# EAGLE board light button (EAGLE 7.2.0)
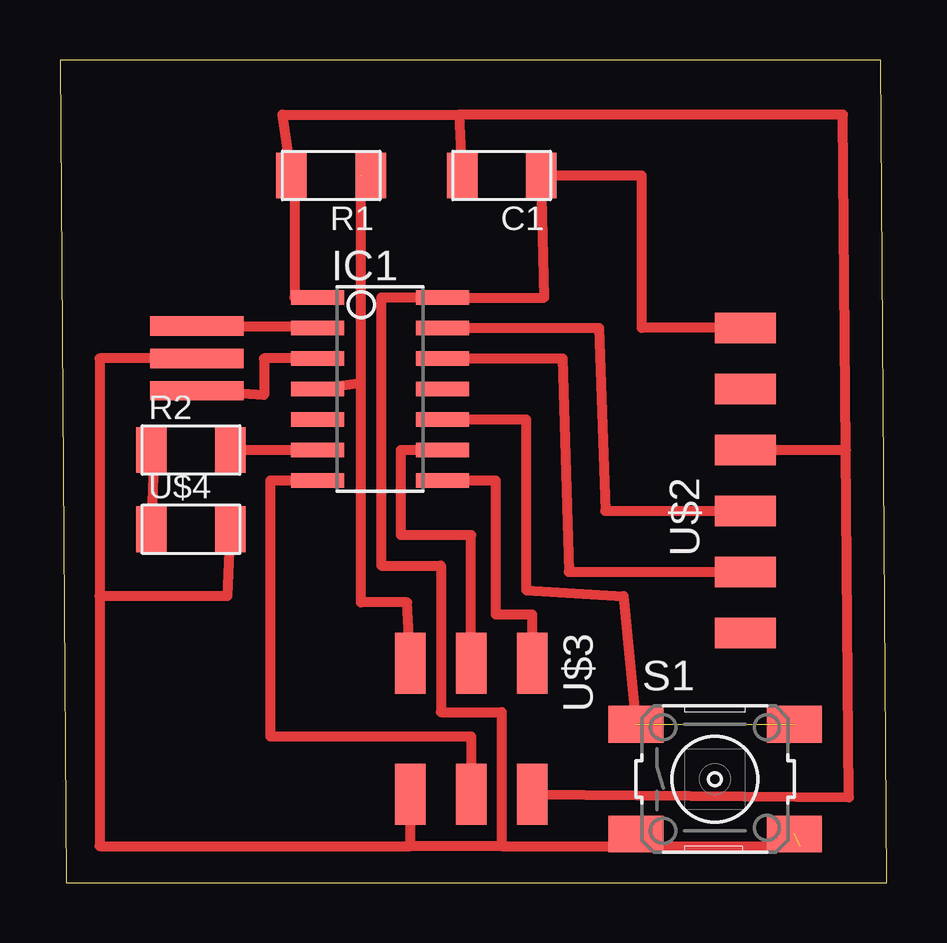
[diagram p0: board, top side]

Size 34.47 x 34.28 mm. Coordinates in mm from the lower left corner, seen from the top.
Outline: 0.25,0 34.47,0 34.21,34.28 0,34.28 0.25,0
Copper layers (1*16): Top 0.035mm / dielectric 1.5mm / Bottom 0.035mm
Design rules "default *": minimum track width 10mil, minimum drill 24mil, track to track 0.41mm, track to pad 0.41mm, pad to pad 0.41mm, via to via 0.41mm, smd to smd 8mil, copper to edge 40mil, drill to drill 8mil, minimum pad ring 10mil, minimum via ring 8mil, stop-mask expansion 4mil, vias tented up to drill 0mil, thermal gap 10mil

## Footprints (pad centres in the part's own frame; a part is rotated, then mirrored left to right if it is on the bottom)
C1206FAB = smd 1.27 x 1.905: 1 -1.651,0; 2 1.651,0
SOIC14 = smd 0.61 x 2.21: 1 -3.81,-2.603; 2 -2.54,-2.603; 3 -1.27,-2.603; 4 0,-2.603; 5 1.27,-2.603; 6 2.54,-2.603; 7 3.81,-2.603; 8 3.81,2.603; 9 2.54,2.603; 10 1.27,2.603; 11 0,2.603; 12 -1.27,2.603; 13 -2.54,2.603; 14 -3.81,2.603
R1206FAB = smd 1.27 x 1.905: 1 -1.651,0; 2 1.651,0
6MM_SWITCH = smd 2.286 x 1.524: 1 -3.302,2.286; 2 3.302,2.286; 3 -3.302,-2.286; 4 3.302,-2.286
EFOBM = smd 0.8 x 3.9: 1 -1.35,0; 2 0,0; 3 1.35,0
1X06SMD = smd 2.54 x 1.27: 1 0,6.35; 2 0,3.81; 3 0,1.27; 4 0,-1.27; 5 0,-3.81; 6 0,-6.35
2X03SMD = smd 2.54 x 1.27: 1 -2.54,2.54; 2 2.92,2.54; 3 -2.54,0; 4 2.92,0; 5 -2.54,-2.54; 6 2.92,-2.54
LED1206FAB = smd 1.27 x 1.905: 1 -1.651,0; 2 1.651,0

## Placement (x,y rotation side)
C1  CAP-US1206FAB  [C1206FAB]  18.42,29.46 180 top
IC1  ATTINY44-SSU  [SOIC14]  13.33,20.57 270 top
R1  [R1206FAB]  11.3,29.46 180 top
R2  [R1206FAB]  5.46,18.03 0 top
S1  [6MM_SWITCH]  27.3,4.32 0 top
U$1  RESONATOR  [EFOBM]  5.71,21.84 270 top
U$2  FTDI-SMD-HEADER  [1X06SMD]  28.58,16.76 0 top
U$3  AVRISPSMD  [2X03SMD]  17.14,6.6 270 top
U$4  LEDFAB1206  [LED1206FAB]  5.46,14.73 0 top

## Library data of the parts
C1 IC1 R1 R2 S1 U$1-U$4 = fab

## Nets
BUTTON: IC1.10 S1.1 S1.2
GND: C1.1 IC1.14 S1.3 S1.4 U$1.2 U$2.1 U$3.6 U$4.2
N$1: IC1.4 R1.1 U$3.5
N$2: IC1.9 U$3.3
N$3: IC1.13 U$2.4
N$4: IC1.12 U$2.5
N$5: IC1.8 U$3.1
N$6: IC1.3 U$1.3
N$7: IC1.7 U$3.4
N$8: IC1.2 U$1.1
N$9: IC1.6 R2.2
N$11: R2.1 U$4.1
VCC: C1.2 IC1.1 R1.2 U$2.3 U$3.2

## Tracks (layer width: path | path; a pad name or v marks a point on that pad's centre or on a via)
BUTTON  (1 unrouted)
  Top 0.406: IC1.10 19.43,19.3 19.43,12.19 23.5,11.94 S1.1
GND  (1 unrouted)
  Top 0.406: U$1.2 1.65,21.84 1.65,11.94 | 1.65,11.94 1.65,1.52 14.61,1.52 | 14.61,1.52 U$3.6 | 16.89,24.38 IC1.14 | IC1.14 13.39,24.38 13.39,13.21 15.88,13.21 15.88,7.11 18.42,7.11 18.42,1.52 | 18.42,1.52 14.61,1.52 | IC1.14 20.19,24.38 C1.1 24.26,29.46 24.26,23.11 U$2.1 | 1.65,11.94 6.98,11.94 U$4.2 | 18.42,1.52 24,1.52 | 24,1.52 30.86,1.52 | S1.3 24,1.52
N$1  (1 unrouted)
  Top 0.406: R1.1 12.55,29.46 | 12.55,29.46 12.52,29.46 | U$3.5 14.48,11.68 12.55,11.68 12.55,20.83 | 12.55,20.83 12.55,29.46 | IC1.4 12.55,20.83
N$2
  Top 0.406: U$3.3 17.14,14.48 14.21,14.48 14.21,18.03 IC1.9
N$3
  Top 0.406: IC1.13 22.48,23.11 22.73,15.49 U$2.4
N$4
  Top 0.406: IC1.12 20.96,21.84 21.21,12.95 U$2.5
N$5
  Top 0.406: IC1.8 18.16,16.76 18.16,11.18 19.69,11.18 U$3.1
N$6
  Top 0.406: IC1.3 8.51,21.84 8.51,20.32 U$1.3
N$7
  Top 0.406: IC1.7 8.76,16.76 8.76,6.1 17.14,6.1 U$3.4
N$8
  Top 0.406: U$1.1 10.79,23.19 10.79,23.11 IC1.2
N$9
  Top 0.406: R2.2 IC1.6
N$11
  Top 0.406: R2.1 3.94,18.03 U$4.1
VCC
  Top 0.406: 16.64,32 9.27,32 R1.2 9.78,29.46 9.78,24.38 IC1.1 | 16.64,32 C1.2 | 32.77,18.04 32.89,3.56 U$3.2 19.69,3.05 | 32.77,18.04 32.64,32 16.64,32 | U$2.3 32.77,18.04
